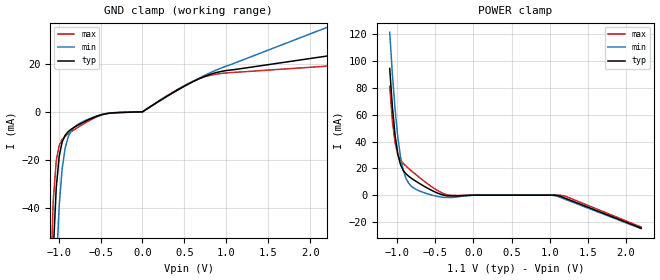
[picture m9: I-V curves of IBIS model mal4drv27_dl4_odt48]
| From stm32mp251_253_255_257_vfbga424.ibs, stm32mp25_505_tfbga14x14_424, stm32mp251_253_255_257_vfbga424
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[Model] mal4drv27_dl4_odt48
Model_type   Input
Polarity   Non-Inverting
Enable   Active-High
C_comp   1.542pF   1.514pF   1.572pF
C_comp_power_clamp   893.006fF   868.450fF   916.252fF
C_comp_gnd_clamp 544.021fF   537.729fF   565.749fF
Vinh = 407.000mV
Vinl = 287.000mV
[Model Spec]
D_overshoot_ampl_h 0.3 NA   NA
D_overshoot_ampl_l 0.3 NA   NA
D_overshoot_area_l 100.000m NA   NA
D_overshoot_area_h 100.000m NA   NA
[Receiver Thresholds]
Vth = 347.000mV
Vth_min = 335.000mV
Vth_max = 369.000mV
Vinh_ac = 600.000mV
Vinh_dc = 600.000mV
Vinl_ac = -600.000mV
Vinl_dc = -600.000mV
Tslew_ac = 5.000ns
Threshold_sensitivity = 0.5
Reference_supply Power_clamp_ref
[Temperature Range]   25.000   125.000   -40.000
[Voltage Range]   1.100V   1.060V   1.170V
[GND Clamp Reference]   0.00V   0.00V   0.00V
[C Comp Corner]
| variable   typ   min   max
C_comp 1.542pF   1.514pF   1.572pF
C_comp_pullup 893.006fF   868.450fF   916.252fF
C_comp_pulldown 544.021fF   565.749fF   537.729fF
[POWER Clamp Reference]   1.100V   1.060V   1.170V
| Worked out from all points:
|   GND clamp passes 1 mA (typ) near -0.46 V on its own axis
|   POWER clamp passes 1 mA (typ) near -0.45 V on its own axis
[GND Clamp]
-1.099V   -106.3mA   -164.1mA   -75.83mA
-1.064V   -59.01mA   -106.6mA   -37.39mA
-1.028V   -31.82mA   -65.58mA   -20.42mA
-992.7mV  -18.55mA   -39.16mA   -14.09mA
-957.3mV  -12.57mA   -23.71mA   -11.56mA
-921.8mV  -9.808mA   -15.2mA    -10.21mA
-886.4mV  -8.315mA   -10.61mA   -9.221mA
-815.5mV  -6.508mA   -6.505mA   -7.526mA
-460.9mV  -963.3uA   -949.5uA   -1.061mA
-1.5uV    -18.58uA   -12.48uA   -23.06uA
780mV     15.31mA    15.88mA    15.01mA
2.198V    23.3mA     35.26mA    19.09mA
[Power Clamp]
-1.098V   94.6mA     121.5mA    81.27mA
-1.063V   65.74mA    90.13mA    55.13mA
-1.027V   44.32mA    63.84mA    38.75mA
-991.8mV  30.54mA    43.23mA    30.36mA
-956.4mV  22.76mA    28.39mA    26.22mA
-885.5mV  15.96mA    12.58mA    21.71mA
-814.5mV  12.63mA    6.678mA    18.17mA
-495.5mV  2.142mA    -675.3uA   4.313mA
-318.2mV  -577.4uA   -1.744mA   -28.48uA
1.029V    -5.796nA   -49.34uA   -750.5pA
1.206V    -2.371mA   -3.205mA   -820.4uA
2.199V    -24.68mA   -25.03mA   -23.85mA
